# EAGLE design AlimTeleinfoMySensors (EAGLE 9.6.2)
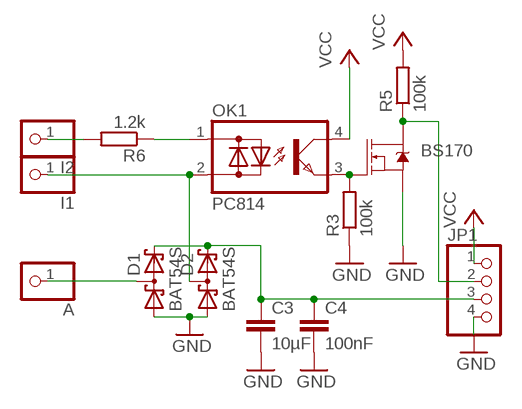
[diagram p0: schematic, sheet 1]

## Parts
A  PINHD-1X1  [1X01]
BS170  MOSFET-NCH-BSS138  [SOT23-3]
C3  10µF  C-EUC1210  [C1210]
C4  100nF  C-EUC1206  [C1206]
D1  BAT54S  [SOT23]
D2  BAT54S  [SOT23]
I1  PINHD-1X1  [1X01]
I2  PINHD-1X1  [1X01]
JP1  PINHD-1X4  [1X04]
OK1  PC814  [DIL04]
R3  100k  R-EU_M1206  [M1206]
R5  100k  R-EU_M1206  [M1206]
R6  1.2k  R-EU_M1206  [M1206]

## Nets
GND: BS170.2(S) C3.2 C4.2 D1.1(A1) D2.1(A1) JP1.4 R3.1
N$8: I2.1 R6.2
N$9: D2.3(C1A2) I1.1 OK1.2(AC2)
N$10: BS170.3(D) JP1.2 R5.1
N$11: C3.1 C4.1 D1.2(C2) D2.2(C2) JP1.3
N$13: OK1.1(AC1) R6.1
N$14: BS170.1(G) OK1.3(E) R3.2
N$15: A.1 D1.3(C1A2)
VCC: JP1.1 OK1.4(C) R5.2

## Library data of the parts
A I1 I2 = pinhead:PINHD-1X1: PIN HEADER
BS170 = SparkFun-DiscreteSemi:MOSFET-NCH: N-channel MOSFETs Voltage controlled devices that allow control of high current outputs. SparkFun Products: SparkFun OpenScale SparkFun Digital Sandbox SparkFun Monster Moto Shield SparkFun MOSFET Power Controller; PROD_ID: TRANS-00830; VALUE: 220mA/50V/3.5Ω
C3 C4 = rcl:C-EU: CAPACITOR, European symbol
D1 D2 = diode:BAT54S: Schottky Diodes Pin connection corrected 2011-05-04 Source: Fairchild .. BAT54.pdf
JP1 = pinhead:PINHD-1X4: PIN HEADER
OK1 = optocoupler:PC814: SHARP OPTO COUPLER; OC_FARNELL: 9707662; OC_NEWARK: unknown
R3 R5 R6 = rcl:R-EU_: RESISTOR, European symbol

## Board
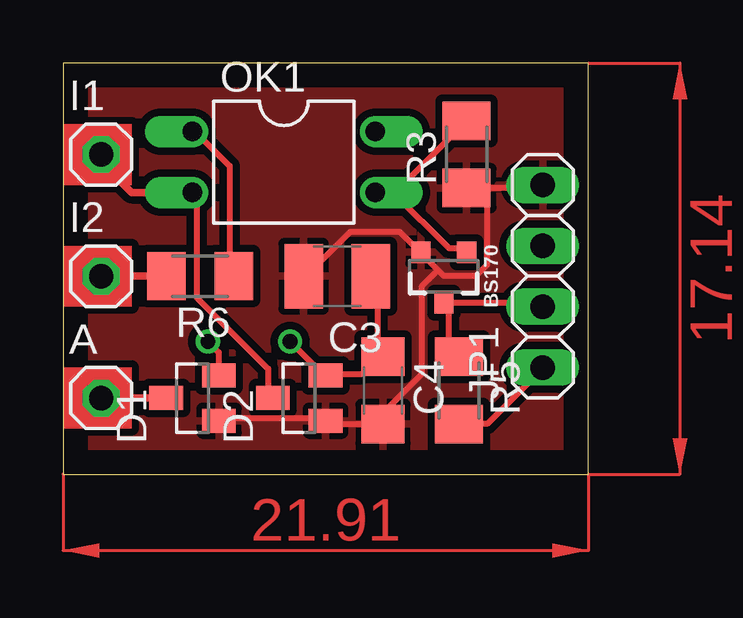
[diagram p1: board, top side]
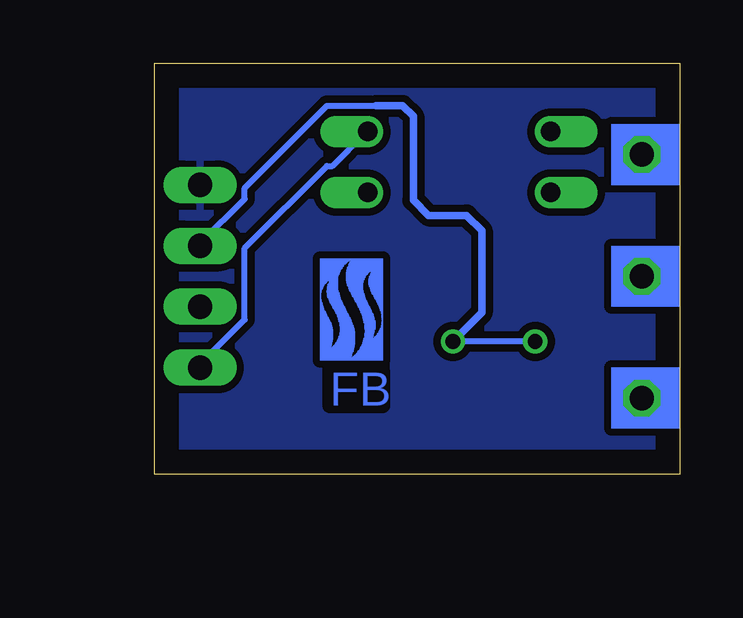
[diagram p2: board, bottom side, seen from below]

Size 21.89 x 17.13 mm. Coordinates in mm from the lower left corner, seen from the top.
Outline: 0,0 21.9,0 21.9,17.13 0,17.13 0,0
Copper layers (1*16): Top 0.035mm / dielectric 1.5mm / Bottom 0.035mm
Design rules "default": minimum track width 10mil, minimum drill 24mil, track to track 8mil, track to pad 8mil, pad to pad 8mil, via to via 8mil, smd to smd 8mil, copper to edge 40mil, drill to drill 8mil, minimum pad ring 10mil, minimum via ring 8mil, stop-mask expansion 4mil, vias tented up to drill 0mil, thermal gap 10mil

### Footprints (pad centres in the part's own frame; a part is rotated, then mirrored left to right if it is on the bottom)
1X01 = drill 1.016 octagon: 1 0,0
SOT23-3 = smd 0.8 x 0.9: 1 -0.95,-1; 2 0.95,-1; 3 0,1.1
C1210 = smd 1.6 x 2.7: 1 -1.4,0; 2 1.4,0
C1206 = smd 1.6 x 1.8: 1 -1.4,0; 2 1.4,0
SOT23 = smd 1 x 1.4: 1 -0.95,-1.1; 2 0.95,-1.1; 3 0,1.1
1X04 = drill 1.016 long: 1 -3.81,0; 2 -1.27,0; 3 1.27,0; 4 3.81,0
DIL04 = drill 0.813 offset: 1 -1.27,-3.81; 2 1.27,-3.81; 3 1.27,3.81; 4 -1.27,3.81
M1206 = smd 1.6 x 2: 1 -1.4,0; 2 1.4,0

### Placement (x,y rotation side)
A  1.59,3.17 0 top
BS170  15.88,8.26 180 top
C3  11.43,8.26 180 top
C4  13.34,3.49 270 top
D1  5.4,3.17 90 top
D2  9.84,3.17 90 top
I1  1.59,13.34 0 top
I2  1.59,8.26 0 top
JP1  20,8.26 90 top
OK1  9.21,13.02 270 top
R3  16.83,13.34 90 top
R5  16.51,3.49 270 top
R6  5.71,8.26 180 top
U$1  [FB]  12.38,4.76 0 top

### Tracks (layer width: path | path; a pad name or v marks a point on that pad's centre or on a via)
GND
  Top 0.254: D1.1 6.72,2.34 10.83,2.34 D2.1 11.06,2.11 13.12,2.11 C4.2 13.35,2.11 13.35,2.57 14.95,4.17 14.95,7.82 15.63,8.51 | 17.69,11.94 19.98,11.94 JP1.4 | 17.69,11.94 17.01,11.94 R3.1 17.69,11.94 | C3.2 10.15,8.28 11.98,10.11 14.03,10.11 14.72,9.42 BS170.2 14.95,9.2 15.63,8.51 | 17.69,11.94 17.69,8.74 17.23,8.28 15.86,8.28 15.63,8.51
  pour Bottom (isolate 0.305): 0,17.14 21.91,17.14 21.91,0 0,0
  pour Top (isolate 0.305): 0,17.14 21.91,17.14 21.91,0 0,0
N$8
  Top 0.305: I2.1 R6.2
N$9
  Top 0.254: D2.3 8.55,3.25 8.55,4.39 5.58,7.37 5.58,11.71 OK1.2
  Top 0.305: I1.1 1.59,13.02 2.86,11.75 OK1.2
N$10
  Top 0.254: 16.09,7.14 16.09,5.31 16.32,5.08 R5.1 | 16.09,7.14 19.98,7.14 JP1.2 | 16.09,7.14 BS170.3
N$11  (via drill 0.61)
  Top 0.254: C3.1 12.89,8.05 13.12,7.82 13.12,5.08 C4.1 13.12,4.85 12.43,4.17 11.06,4.17 D2.2 10.83,4.17 v9.46,5.54 | v6.03,5.54 6.49,5.08 6.49,4.17 D1.2
  Bottom 0.254: 12.66,15.37 14.72,15.37 18.15,11.94 18.15,11.48 19.98,9.65 JP1.3 | v6.03,5.54 v9.46,5.54
  Bottom 0.305: 12.66,15.37 11.56,15.37 11.11,14.92 11.11,11.43 10.48,10.79 8.89,10.79 8.26,10.16 8.26,6.74 v9.46,5.54
N$13
  Top 0.254: R6.1 6.95,8.28 6.95,12.85 5.58,14.22 OK1.1
N$14
  Top 0.254: 13.8,11.71 16.09,9.42 16.78,9.42 BS170.1 | 13.8,11.71 13.12,11.71 OK1.3 13.8,11.71 | 13.8,11.71 16.78,14.68 R3.2
N$15
  Top 0.305: A.1 D1.3
VCC
  Top 0.254: R5.2 16.55,2.11 17.69,2.11 19.98,4.39 JP1.1
  Bottom 0.254: OK1.4 13.12,14.22 14.49,12.85 14.72,12.85 18.15,9.42 18.15,6.45 19.98,4.62 JP1.1
(copper drawn outside any net)
  shapes: Bottom area x3, Top area x5

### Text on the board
Bottom: FB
